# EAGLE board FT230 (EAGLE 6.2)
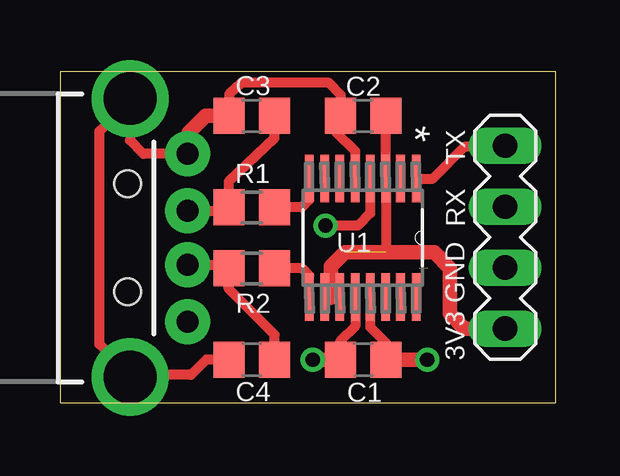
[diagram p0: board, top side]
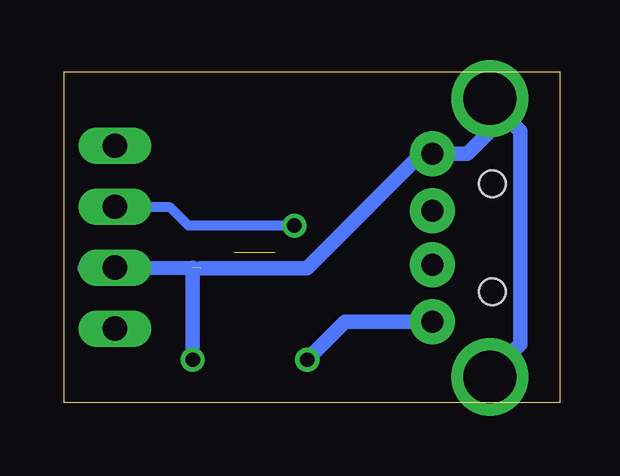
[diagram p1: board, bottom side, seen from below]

Size 20.68 x 13.79 mm. Coordinates in mm from the lower left corner, seen from the top.
Outline: 0,0 20.68,0 20.68,13.79 0,13.79 0,0
Copper layers (1*16): Top 0.035mm / dielectric 1.5mm / Bottom 0.035mm
Design rules: minimum track width 10mil, minimum drill 24mil, track to track 8mil, track to pad 8mil, pad to pad 8mil, via to via 8mil, smd to smd 8mil, copper to edge 40mil, drill to drill 8mil, minimum pad ring 10mil, minimum via ring 8mil, stop-mask expansion 4mil, vias tented up to drill 0mil, thermal gap 10mil

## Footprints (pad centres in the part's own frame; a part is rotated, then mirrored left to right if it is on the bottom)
C0805 = smd 1.3 x 1.5: 1 -0.95,0; 2 0.95,0
R0805 = smd 1.3 x 1.5: 1 -0.95,0; 2 0.95,0
MA04-1 = drill 1.016 long: 1 -3.81,0; 2 -1.27,0; 3 1.27,0; 4 3.81,0
SOP63P600X175-16N = smd 1.981 x 0.356: 1 -2.464,2.235; 2 -2.464,1.575; 3 -2.464,0.965; 4 -2.464,0.305; 5 -2.464,-0.305; 6 -2.464,-0.965; 7 -2.464,-1.575; 8 -2.464,-2.235; 9 2.464,-2.235; 10 2.464,-1.575; 11 2.464,-0.965; 12 2.464,-0.305; 13 2.464,0.305; 14 2.464,0.965; 15 2.464,1.575; 16 2.464,2.235
USB-A-H = drill 0.914 pad 1.88: D+ 2.4,1.127; D- 2.4,-1.127; GND 2.4,3.5; VBUS 2.4,-3.5 | drill 2.2: GND@1 0,5.8; GND@2 0,-5.8 | hole 1.1: -0.1,2.25; -0.1,-2.25

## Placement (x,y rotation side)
C1  [C0805]  12.65,1.8 0 top
C2  [C0805]  12.65,11.96 180 top
C3  [C0805]  8,11.96 180 top
C4  [C0805]  8,1.8 180 top
R1  [R0805]  8,8.15 0 top
R2  [R0805]  8,5.61 0 top
SV1  [MA04-1]  18.57,6.91 270 top
U1  FT230XS  [SOP63P600X175-16N]  12.62,6.88 270 top
X1  USB-A-H  [USB-A-H]  2.92,6.88 0 top

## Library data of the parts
C1-C4 R1 R2 = rcl
SV1 = con-lstb; OC_FARNELL: unknown; OC_NEWARK: unknown
U1 = zilog; MPN: FT230XS; OC_FARNELL: 2081321; OC_NEWARK: 83T7087; PACKAGE: SSOP-16; SUPPLIER: FTDI
X1 = moja

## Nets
3V3: C2.1 SV1.4 U1.3 U1.10 U1.11
CB0: U1.15
CB1: U1.14
CB2: U1.7
CB3: U1.16
CTS: U1.6
N$1: C3.1 R1.1 X1.D+
N$2: C4.1 R2.1 X1.D-
N$3: R1.2 U1.8
N$4: R2.2 U1.9
N$6: C1.1 U1.12 X1.VBUS
N$7: SV1.1 U1.1
N$16: C1.2 C2.2 C3.2 C4.2 SV1.3 U1.5 U1.13 X1.GND
RXD: SV1.2 U1.4

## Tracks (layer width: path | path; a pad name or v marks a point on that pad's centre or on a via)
3V3  (1 unrouted)
  Top 0.406: C2.1 13.59,12.48 U1.3 13.59,6.27 | 11.3,4.39 11.18,4.39 U1.11 U1.10
  Top 0.61: SV1.4 16.87,3.1 16.26,3.71 16.26,5.61 15.62,6.27 13.59,6.27 11.89,6.27 11.3,5.69 11.3,4.39
N$1
  Top 0.406: X1.D+ 7.05,8.01 R1.1 7.05,9.24 8.94,11.02 C3.1
N$2
  Top 0.406: X1.D- 6.42,5.76 R2.1 7.04,5.6 7.04,4.75 8.95,2.83 C4.1
N$3
  Top 0.406: U1.8 10.39,8.46 10.08,8.15 R1.2
N$4
  Top 0.406: U1.9 10.39,5.31 10.08,5.61 R2.2
N$6  (via drill 0.6)
  Top 0.406: U1.12 12.32,3.2 11.68,2.57 11.68,1.26 C1.1
  Top 0.61: v10.54,1.8 C1.1
  Bottom 0.61: X1.VBUS 8.96,3.38 v10.54,1.8
N$7
  Top 0.406: U1.1 15.54,9.35 16.89,10.69 19.81,10.69 SV1.1
N$16  (via drill 0.6)  (1 unrouted)
  Top 0.406: U1.13 12.93,3.18 13.59,2.51 13.61,1.64 C1.2 | U1.5 12.32,10.49 11.53,11.25 11.53,11.93 C2.2 11.71,12.83 11.23,13.34 7.54,13.34 7.06,12.88 C3.2 | C4.2 6.1,1.8 5.46,1.17 2.92,1.17 1.65,2.44 1.65,11.33 2.92,12.6 2.92,10.95 3.47,10.38 X1.GND
  Top 0.61: C1.2 v15.32,1.8 | C3.2 6.07,11.96 5.36,11.25 5.36,10.45 X1.GND
  Bottom 0.61: v15.32,1.8 15.32,5.64 19.81,5.61 SV1.3 | 2.92,1.17 1.65,2.44 1.65,11.33 2.92,12.6 2.92,11.33 3.87,10.38 X1.GND 5.8,10.36 10.54,5.61 14.99,5.61
RXD  (via drill 0.6)
  Top 0.406: U1.4 12.93,7.9 12.42,7.39 v11.07,7.39
  Bottom 0.406: v11.07,7.39 15.49,7.39 16.26,8.15 18.54,8.15 SV1.2

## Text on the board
tNames: TX | RX | GND | 3V3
